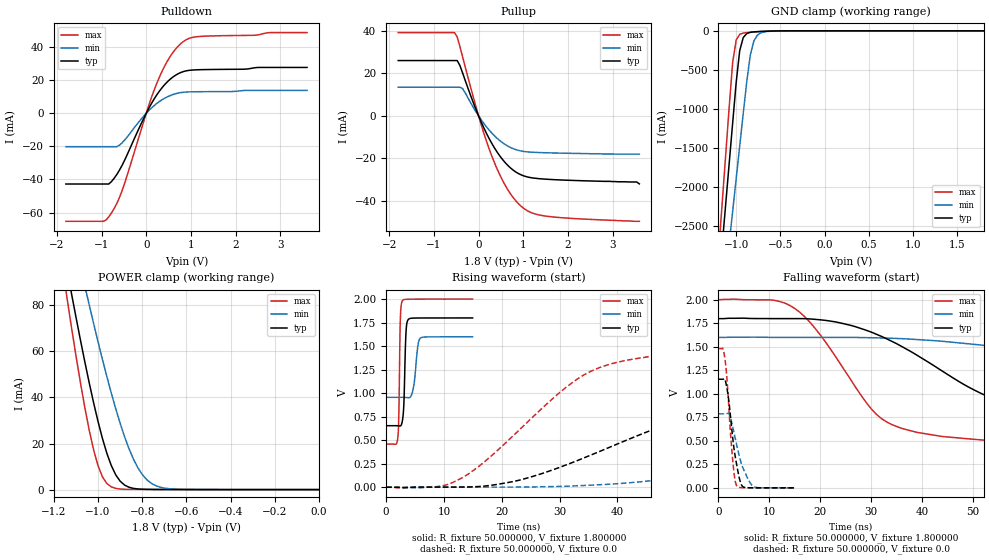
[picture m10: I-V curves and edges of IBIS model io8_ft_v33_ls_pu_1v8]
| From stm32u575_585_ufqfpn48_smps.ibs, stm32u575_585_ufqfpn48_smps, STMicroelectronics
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|   Model io8_ft_v33_ls_pu_1v8
[Model]  io8_ft_v33_ls_pu_1v8
Model_type I/O
Polarity   Non-Inverting
Enable   Active-Low
Vinl =   0.540000V
Vinh =   1.260000V
Vmeas =  0.900000V
Cref =   50.000000pF
Rref =   100.000000M
Vref =   0.0V
C_comp   3.087500pF   3.086600pF   3.135700pF
[Temperature Range]   25.000000   0.140000k   -40.000000
[Pullup Reference]   1.800000V   1.600000V   2.000000V
[Pulldown Reference]   0.0V   0.0V   0.0V
[POWER Clamp Reference]   1.800000V   1.600000V   2.000000V
[GND Clamp Reference]   0.0V   0.0V   0.0V
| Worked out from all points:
|   slope of the pulldown table from 0 to 0.27 V, typ, clamps not added: 21.7 ohm
|   slope of the pullup table from 0 to 0.27 V, typ, clamps not added: 22.6 ohm
|   GND clamp passes 1 mA (typ) near -0.51 V on its own axis
|   POWER clamp passes 1 mA (typ) near -0.86 V on its own axis
|   rising waveform, R_fixture 50.000000, V_fixture 1.800000: 20-80 % time 315ps typ, 629ps min, 225ps max; typ from 0.655 V to 1.8 V
|   rising waveform, R_fixture 50.000000, V_fixture 0.0: 20-80 % time 31.3ns typ, 66.7ns min, 16.5ns max; typ from 0.001 V to 1.16 V
|   falling waveform, R_fixture 50.000000, V_fixture 1.800000: 20-80 % time 24.6ns typ, 55.4ns min, 12.3ns max; typ from 1.8 V to 0.655 V
|   falling waveform, R_fixture 50.000000, V_fixture 0.0: 20-80 % time 1.6ns typ, 2.38ns min, 1.17ns max; typ from 1.16 V to 0.001 V
[Pulldown]
|Voltage   I(typ)   I(min)   I(max)
-1.8V     -42.74mA   -20.21mA   -65.25mA
-960mV    -42.74mA   -20.21mA   -65.25mA
-780mV    -41.3mA    -20.21mA   -60.25mA
-660mV    -37mA      -20.2mA    -54.5mA
-540mV    -31.39mA   -17.82mA   -46.65mA
0V        0A         0A         0A
240mV     11.28mA    6.002mA    18.38mA
480mV     19.17mA    10.02mA    31.83mA
780mV     24.67mA    12.5mA     42.21mA
960mV     25.9mA     12.9mA     45.21mA
1.2V      26.29mA    13.01mA    46.37mA
3.6V      27.66mA    13.81mA    48.71mA
[Pullup]
|Voltage   I(typ)   I(min)   I(max)
-1.8V     26.06mA    13.5mA     39.23mA
-540mV    26.06mA    13.5mA     39.23mA
-480mV    26.06mA    13.5mA     37.18mA
-360mV    20.34mA    12.93mA    27.94mA
0V        590fA      222pA      10fA
300mV     -13.1mA    -8.158mA   -19.11mA
480mV     -18.98mA   -11.71mA   -27.97mA
660mV     -23.42mA   -14.29mA   -34.95mA
1.02V     -28.29mA   -16.75mA   -43.65mA
1.26V     -29.33mA   -17.15mA   -46.11mA
1.62V     -29.92mA   -17.41mA   -47.45mA
3.6V      -32mA      -18mA      -49.6mA
[GND_clamp]
|Voltage   I(typ)   I(min)   I(max)
-1.8V     -9.707A    -9.942A    -9.774A
-1.2V     -3.309A    -4.006A    -2.864A
-1.16V    -2.777A    -3.584A    -2.239A
-1.12V    -2.246A    -3.162A    -1.614A
-1.04V    -1.186A    -2.319A    -408.6mA
-1V       -663.9mA   -1.898A    -117.8mA
-960mV    -254mA     -1.478A    -45.14mA
-920mV    -86.03mA   -1.06A     -28.58mA
-840mV    -19.12mA   -308.9mA   -18.74mA
-800mV    -13.39mA   -130.8mA   -15.31mA
-720mV    -7.948mA   -25.37mA   -9.381mA
1.8V      0A         14.97nA    0A
[POWER_clamp]
|Voltage   I(typ)   I(min)   I(max)
-1.8V     470.9mA    433.7mA    554.6mA
-1.14V    95.29mA    122.7mA    82.89mA
-1.12V    85mA       114mA      70.34mA
-1.06V    55.55mA    88.43mA    35.74mA
-1.04V    46.38mA    80.17mA    25.83mA
-1V       29.54mA    64.14mA    10.37mA
-940mV    10.43mA    41.88mA    1.179mA
-900mV    3.662mA    28.79mA    252.8uA
-840mV    528.6uA    13.26mA    97.33uA
-800mV    159uA      6.55mA     88.9uA
-740mV    60.12uA    1.751mA    70.99uA
0V        0A         18.15nA    0A
[Ramp]
| variable   typ   min   max
dV/dt_r  0.69287/31.26590n   0.47197/66.66988n   0.88855/16.41682n
dV/dt_f  0.68716/24.57820n   0.38639/55.33754n   0.92439/12.27200n
R_load = 50.000000
[Rising Waveform]
R_fixture= 50.000000
V_fixture= 1.800000
V_fixture_min= 1.600000
V_fixture_max= 2.000000
|time   V(typ)   V(min)   V(max)
0s        654.8mV    956mV      459.3mV
2.012ns   654.2mV    956.1mV    525.3mV
2.192ns   653mV      956.1mV    778.8mV
2.462ns   652.4mV    956.1mV    1.804V
2.793ns   701.5mV    956mV      1.981V
3.063ns   886.4mV    955.8mV    1.994V
3.423ns   1.636V     954.7mV    1.998V
3.814ns   1.783V     952.3mV    1.999V
5.856ns   1.799V     1.582V     2V
14.95ns   1.8V       1.6V       2V
[Rising Waveform]
R_fixture= 50.000000
V_fixture= 0.0
V_fixture_min= 0.0
V_fixture_max= 0.0
|time   V(typ)   V(min)   V(max)
0s        611.3uV    688.3uV    577.8uV
13.01ns   3.025mV    1.558mV    96.43mV
23.02ns   75.7mV     2.58mV     609.5mV
36.04ns   358.5mV    24.72mV    1.251V
58.06ns   861.6mV    159.6mV    1.449V
72.07ns   1.027V     279.3mV    1.47V
90.09ns   1.106V     428mV      1.478V
130.1ns   1.148V     652.5mV    1.482V
167.2ns   1.154V     738mV      1.482V
498.5ns   1.155V     787.4mV    1.482V
[Falling Waveform]
R_fixture= 50.000000
V_fixture= 1.800000
V_fixture_min= 1.600000
V_fixture_max= 2.000000
|time   V(typ)   V(min)   V(max)
0s        1.8V       1.6V       2V
11.01ns   1.8V       1.6V       1.994V
15.02ns   1.8V       1.6V       1.907V
33.03ns   1.586V     1.593V     701.8mV
52.05ns   993.6mV    1.516V     508.7mV
63.06ns   828.3mV    1.433V     484.5mV
80.08ns   733.2mV    1.27V      468.5mV
107.1ns   681.8mV    1.107V     461.4mV
150.2ns   660.7mV    1.013V     459.4mV
498.5ns   654.8mV    956mV      459.3mV
[Falling Waveform]
R_fixture= 50.000000
V_fixture= 0.0
V_fixture_min= 0.0
V_fixture_max= 0.0
|time   V(typ)   V(min)   V(max)
0s        1.155V     787.4mV    1.482V
840.8ps   1.155V     787.4mV    1.482V
1.291ns   1.15V      787.2mV    1.364V
2.012ns   932mV      790.5mV    875mV
2.763ns   548mV      657.3mV    314.8mV
3.153ns   379.1mV    561.8mV    116.2mV
3.514ns   265.9mV    472.1mV    28.18mV
4.685ns   17.77mV    229.6mV    2.442mV
6.607ns   1.304mV    26.72mV    1.116mV
14.95ns   611.3uV    688.3uV    577.8uV
